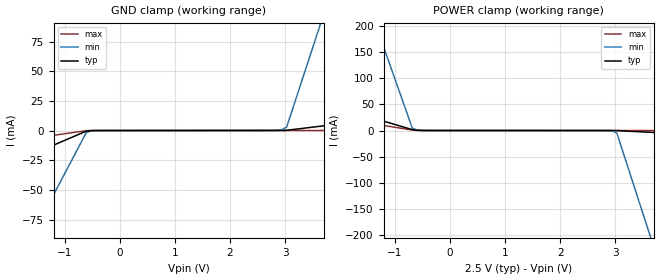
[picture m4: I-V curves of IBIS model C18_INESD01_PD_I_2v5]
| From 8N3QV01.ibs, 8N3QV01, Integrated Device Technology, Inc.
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[Model] C18_INESD01_PD_I_2v5
Model_type   Input
Polarity   Non-Inverting
Vinl = 0.7V
Vinh = 1.7V
|   typ   min   max
C_comp   2pF   1.5pF   2.5pF
|   typ   min   max
[Voltage range]   2.5V   2.375V   2.625V
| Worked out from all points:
|   GND clamp passes 1 mA (typ) near -0.63 V on its own axis
|   POWER clamp passes 1 mA (typ) near -0.63 V on its own axis
[GND_clamp]
|Voltage   I (typ)   I (min)   I (max)
-2.5V     -38.19mA   -169mA     -12.74mA
-1.591V   -20.1mA    -88.72mA   -6.679mA
-1.515V   -18.6mA    -82.03mA   -6.174mA
-606.1mV  -511.5uA   -1.738mA   -108.1uA
-530.3mV  -105.5uA   -396.3uA   -20.16uA
-378.8mV  -9.239uA   -22.06uA   -6.496uA
2.727V    54.52uA    67.84uA    46.41uA
2.955V    75.5uA     941.4uA    50.29uA
3.03V     177.1uA    2.92mA     51.74uA
3.561V    3.18mA     78mA       81.96uA
3.636V    3.609mA    88.72mA    86.28uA
5V        11.33mA    281.8mA    164uA
[Power_clamp]
|Voltage   I (typ)   I (min)   I (max)
-2.5V     58.51mA    546mA      31.95mA
-1.364V   22.98mA    207.7mA    12.47mA
-1.288V   20.61mA    185.1mA    11.17mA
-681.8mV  1.659mA    4.655mA    783.2uA
-606.1mV  606uA      1.384mA    203uA
-454.5mV  75.5uA     144.2uA    53.61uA
2.955V    -23.28uA   -1.039mA   -5.615uA
3.03V     -105.5uA   -4.685mA   -7.036uA
3.561V    -2.948mA   -176.9mA   -30.39uA
3.636V    -3.354mA   -201.5mA   -33.72uA
5V        -10.66mA   -644.3mA   -93.78uA
